(* Logix 5000 AddOnInstructionDefinition export AMP_Hard_Stop_Homing; software revision 20.04 *)

TYPE AMP_Status_Word :   // Applied Motion Input Assembly Status Word
STRUCT
   Enabled : BOOL;   // Motor Enabled (Motor Disabled if this bit = 0)
   Sampling : BOOL;   // Sampling (for Quick Tuner)
   Drive_Fault : BOOL;   // Drive Fault (check Alarm Code)
   In_Position : BOOL;   // In Position (motor is in position)
   Moving : BOOL;   // Moving (motor is moving)
   Jogging : BOOL;   // Jogging (currently in jog mode)
   Stopping : BOOL;   // Stopping (in the process of stopping from a stop command)
   Waiting : BOOL;   // Waiting (for an input; executing a WI command)
   Saving : BOOL;   // Saving (parameter data is being saved)
   Alarm_Present : BOOL;   // Alarm present (check Alarm Code)
   Homing : BOOL;   // Homing (executing an SH command)
   Wait_Time : BOOL;   // Waiting (for time; executing a WD or WT command)
   Wizard_Running : BOOL;   // Wizard running (Timing Wizard is running)
   Checking_Encoder : BOOL;   // Checking encoder (Timing Wizard is running)
   Q_Program_Running : BOOL;   // Q Program is running
   Initializing : BOOL;   // Initializing (happens at power up) ; Servo Ready (for SV200 drives only)
END_STRUCT
END_TYPE

TYPE AMP_Input_Assembly_v2 :   // Applied Motion Drive Input Assembly Version 2.0
STRUCT
   Status_Code : DINT;   // Status Code
   Alarm_Code : DINT;   // Alarm Code
   Voltage : DINT;   // Supply Voltage (x0.1V)
   Current : DINT;   // Actual Current (mA)
   Temp : DINT;   // Drive Temperature (0.1 deg C)
   Encoder_Position : DINT;   // Encoder Position (20,000 counts = 1 shaft turn)
   Absolute_Position : DINT;   // Absolute Position (20,000 counts = 1 shaft turn)
   Position_Error : DINT;   // Position Error (counts)
   Actual_Velocity : DINT;   // Actual Velocity (rev/sec * 240, 0 when no encoder)
   Extended_Inputs : DINT;   // Input Status (Extended)
   Main_Board_Inputs : DINT;   // Input Status (Main board)
   Word11 : DINT;   // Reserved
   Analog_Input_1 : DINT;   // Analog Input 1 (ADC counts, 0=min V, 16383 = max V)
   Analog_Input_2 : DINT;   // Analog Input 2 (ADC counts, 0=min V, 16383 = max V)
END_STRUCT
END_TYPE

ADD_ON_INSTRUCTION AMP_Hard_Stop_Homing   (* revision 1.0 *)
// Applied Motion - Hard Stop Homing AOI
// Help:
// The Hard Stop Homing AOI accepts all the required parameters for SCL commands HV1, HV2, HV3, HA1, HA2, HA3, HL1, HL2, HL3, HC, HD, HO and then sends the HS command to initiate the Hard Stop Homing move.
VAR_IN_OUT
   Input : DINT[14]; {required}   // Drive Input Assembly
   Output : DINT[16]; {required}   // Drive Output Assembly
        [0]   // Command Word
        [1]   // Jog Speed (0.25 rev/min)
        [2]   // Jog Acceleration (10 rev/s/s)
        [3]   // Jog Deceleration (10 rev/s/s)
        [4]   // Point-to-Point Velocity (0.25 rev/min)
        [5]   // Point-to-Point Acceleration (10 rev/s/s)
        [6]   // Point-to-Point Deceleration (10 rev/s/s)
        [7]   // Point-to-Point Distance (Motor steps)
        [9]   // (2x ASCII Letters in 16 lower word)
        [10]   // Data/Register 1
        [11]   // Data/Register 2
END_VAR
VAR_INPUT
   RPI : DINT := 100; {visible}   // Drive Connection Request Packet Interval (milliseconds)
   Start : BOOL; {required}   // Start the Homing
   HV1 : REAL; {required}   // Velocity used while seeking the hard stop (rev/s)
   HV2 : REAL; {required}   // Velocity when moving offset distance set by HO (rev/s)
   HV3 : REAL; {required}   // Velocity when searching for encoder index if desired (rev/s)
   HA1 : REAL; {required}   // Accel used while seeking the hard stop (rev/s/s)
   HA2 : REAL; {required}   // Accel when moving offset distance set by HO (rev/s/s)
   HA3 : REAL; {required}   // Accel when searching for encoder index if desired (rev/s/s)
   HL1 : REAL; {required}   // Decel used while seeking the hard stop (rev/s/s)
   HL2 : REAL; {required}   // Decel when moving offset distance set by HO (rev/s/s)
   HL3 : REAL; {required}   // Decel when searching for encoder index if desired (rev/s/s)
   HC : REAL; {required}   // Hard Stop Current (Amps)
   HD : DINT; {required}   // Hard Stop Fault Delay (ms)
   HO : DINT; {required}   // Home Offset (steps, negative = CCW, positive = CW)
   HS : DINT; {required}   // Hard Stop method (0 = without index, 1 = with index)
END_VAR
VAR_OUTPUT
   Sent : BOOL; {access Read Only, visible}   // All parameter setting and homing commands have been sent to drive
   In_Progress : BOOL; {access Read Only, visible}   // The setting of parameters and/or homing are in progress
   Done : BOOL; {access Read Only, visible}   // Homing Move completed without errors - desired position reached
   Error : BOOL; {access Read Only, visible}   // Homing failed to complete - drive not ready or faulted
   State : DINT := 34; {access Read Only}   // Internal state of progress
END_VAR
VAR
   Loc_StatusCode : AMP_Status_Word;
   Loc_CommandOff_Timer : TIMER;   // Timer to make sure command value was 0 before sending a new command
   Loc_CommandOn_Timer : TIMER;   // Timer to make sure command value is set long enough to be sent to drive
   Loc_Input_Assembly : AMP_Input_Assembly_v2; {access None}
   Loc_Start_ONS : BOOL; {access None}
END_VAR

ROUTINE Logic   (* ladder *)
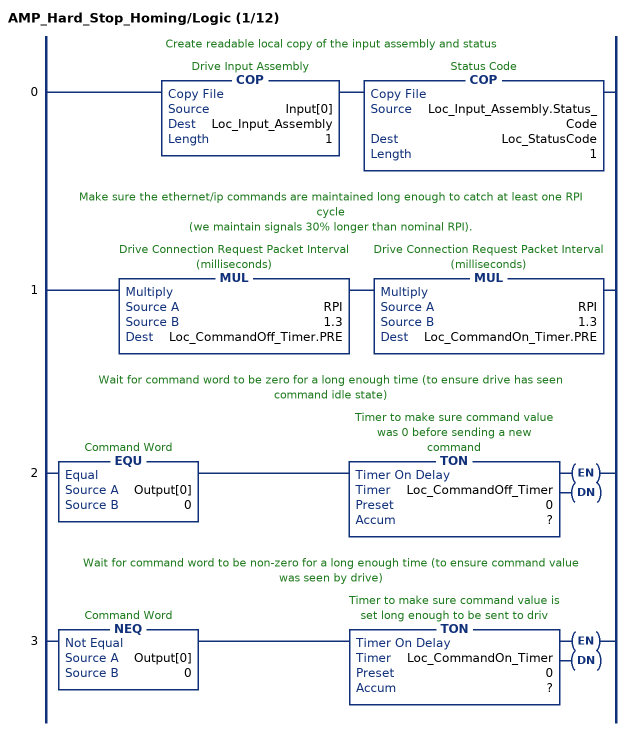
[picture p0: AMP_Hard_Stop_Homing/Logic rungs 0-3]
   // Create readable local copy of the input assembly and status
   0: COP(Input[0],Loc_Input_Assembly,1)COP(Loc_Input_Assembly.Status_Code,Loc_StatusCode,1);
   // Make sure the ethernet/ip commands are maintained long enough to catch at least one RPI cycle
   // (we maintain signals 30% longer than nominal RPI).
   1: MUL(RPI,1.3,Loc_CommandOff_Timer.PRE)MUL(RPI,1.3,Loc_CommandOn_Timer.PRE);
   // Wait for command word to be zero for a long enough time (to ensure drive has seen command idle state)
   2: EQU(Output[0],0)TON(Loc_CommandOff_Timer,?,?);
   // Wait for command word to be non-zero for a long enough time (to ensure command value was seen by drive)
   3: NEQ(Output[0],0)TON(Loc_CommandOn_Timer,?,?);
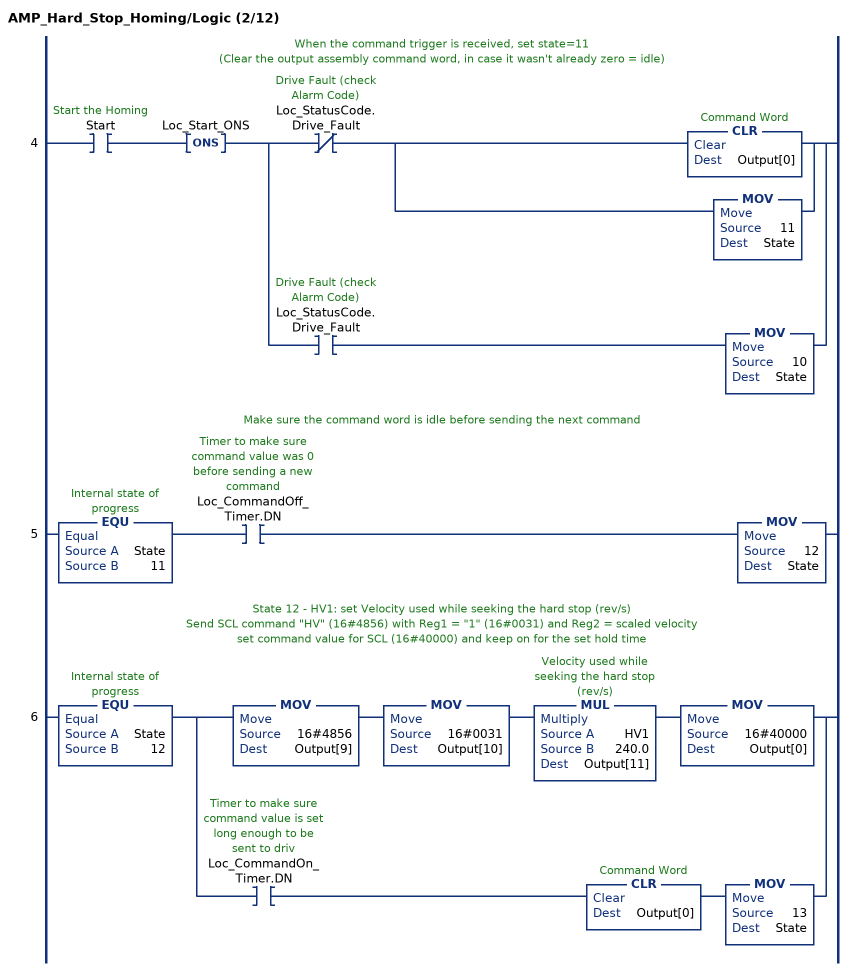
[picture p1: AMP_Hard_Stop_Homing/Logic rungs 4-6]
   // When the command trigger is received, set state=11
   // (Clear the output assembly command word, in case it wasn't already zero = idle)
   4: XIC(Start)ONS(Loc_Start_ONS)[XIO(Loc_StatusCode.Drive_Fault) [CLR(Output[0]) ,MOV(11,State) ] ,XIC(Loc_StatusCode.Drive_Fault) MOV(10,State) ];
   // Make sure the command word is idle before sending the next command
   5: EQU(State,11)XIC(Loc_CommandOff_Timer.DN)MOV(12,State);
   // State 12 - HV1: set Velocity used while seeking the hard stop (rev/s)
   // Send SCL command "HV" (16#4856) with Reg1 = "1" (16#0031) and Reg2 = scaled velocity
   // set command value for SCL (16#40000) and keep on for the set hold time
   6: EQU(State,12)[MOV(16#4856,Output[9]) MOV(16#0031,Output[10]) MUL(HV1,240.0,Output[11]) MOV(16#40000,Output[0]) ,XIC(Loc_CommandOn_Timer.DN) CLR(Output[0]) MOV(13,State) ];
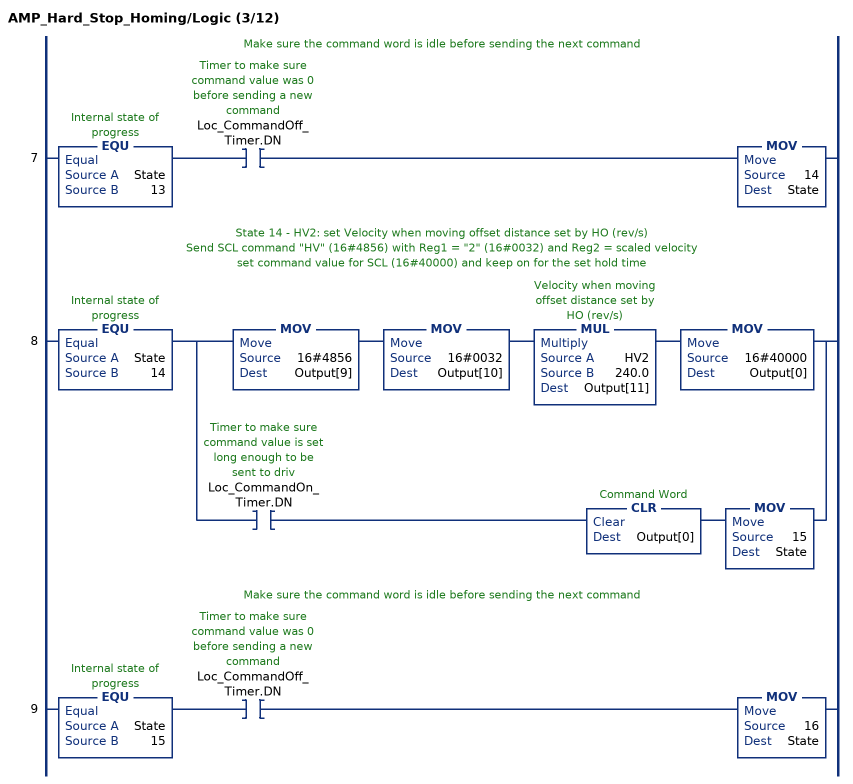
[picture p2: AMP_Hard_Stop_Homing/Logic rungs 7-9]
   // Make sure the command word is idle before sending the next command
   7: EQU(State,13)XIC(Loc_CommandOff_Timer.DN)MOV(14,State);
   // State 14 - HV2: set Velocity when moving offset distance set by HO (rev/s)
   // Send SCL command "HV" (16#4856) with Reg1 = "2" (16#0032) and Reg2 = scaled velocity
   // set command value for SCL (16#40000) and keep on for the set hold time
   8: EQU(State,14)[MOV(16#4856,Output[9]) MOV(16#0032,Output[10]) MUL(HV2,240.0,Output[11]) MOV(16#40000,Output[0]) ,XIC(Loc_CommandOn_Timer.DN) CLR(Output[0]) MOV(15,State) ];
   // Make sure the command word is idle before sending the next command
   9: EQU(State,15)XIC(Loc_CommandOff_Timer.DN)MOV(16,State);
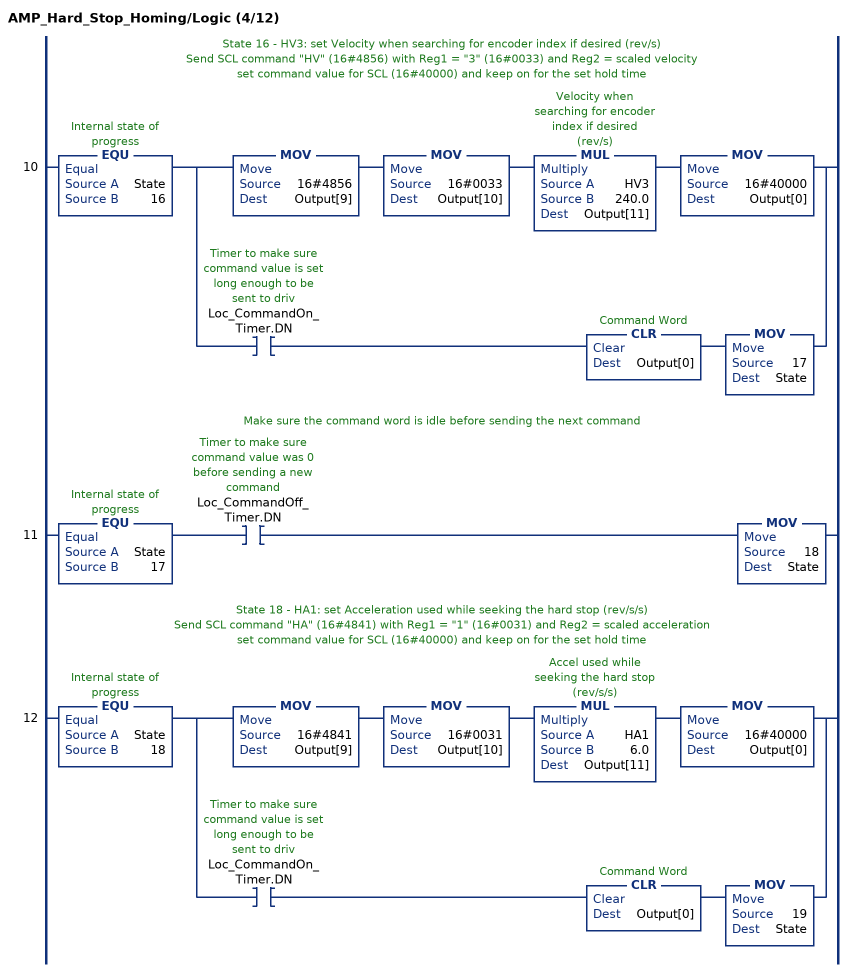
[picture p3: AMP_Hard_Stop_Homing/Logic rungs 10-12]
   // State 16 - HV3: set Velocity when searching for encoder index if desired (rev/s)
   // Send SCL command "HV" (16#4856) with Reg1 = "3" (16#0033) and Reg2 = scaled velocity
   // set command value for SCL (16#40000) and keep on for the set hold time
   10: EQU(State,16)[MOV(16#4856,Output[9]) MOV(16#0033,Output[10]) MUL(HV3,240.0,Output[11]) MOV(16#40000,Output[0]) ,XIC(Loc_CommandOn_Timer.DN) CLR(Output[0]) MOV(17,State) ];
   // Make sure the command word is idle before sending the next command
   11: EQU(State,17)XIC(Loc_CommandOff_Timer.DN)MOV(18,State);
   // State 18 - HA1: set Acceleration used while seeking the hard stop (rev/s/s)
   // Send SCL command "HA" (16#4841) with Reg1 = "1" (16#0031) and Reg2 = scaled acceleration
   // set command value for SCL (16#40000) and keep on for the set hold time
   12: EQU(State,18)[MOV(16#4841,Output[9]) MOV(16#0031,Output[10]) MUL(HA1,6.0,Output[11]) MOV(16#40000,Output[0]) ,XIC(Loc_CommandOn_Timer.DN) CLR(Output[0]) MOV(19,State) ];
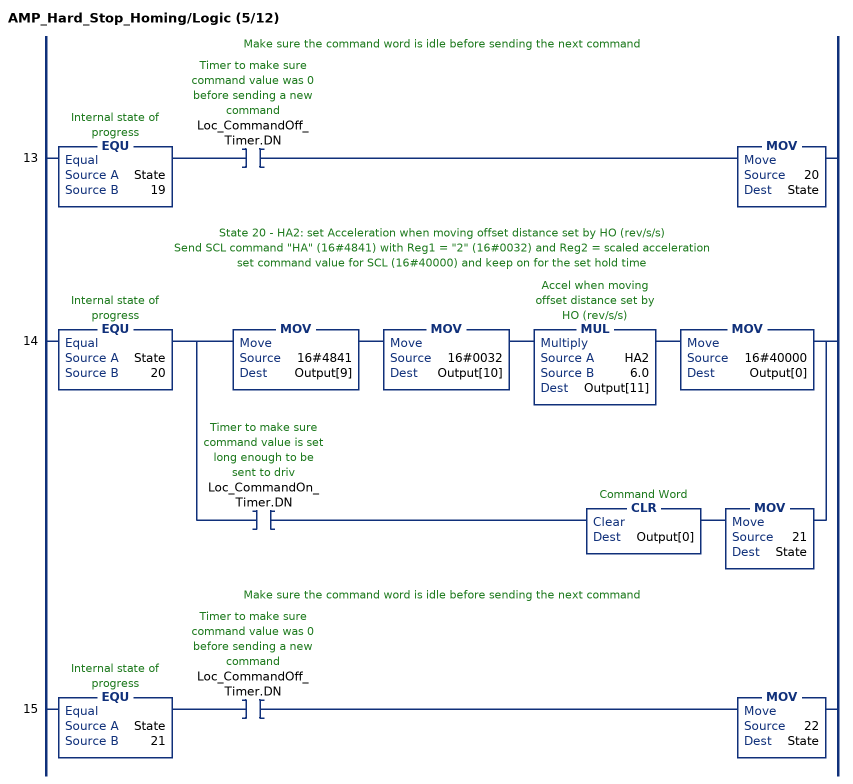
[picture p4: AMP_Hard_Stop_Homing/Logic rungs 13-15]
   // Make sure the command word is idle before sending the next command
   13: EQU(State,19)XIC(Loc_CommandOff_Timer.DN)MOV(20,State);
   // State 20 - HA2: set Acceleration when moving offset distance set by HO (rev/s/s)
   // Send SCL command "HA" (16#4841) with Reg1 = "2" (16#0032) and Reg2 = scaled acceleration
   // set command value for SCL (16#40000) and keep on for the set hold time
   14: EQU(State,20)[MOV(16#4841,Output[9]) MOV(16#0032,Output[10]) MUL(HA2,6.0,Output[11]) MOV(16#40000,Output[0]) ,XIC(Loc_CommandOn_Timer.DN) CLR(Output[0]) MOV(21,State) ];
   // Make sure the command word is idle before sending the next command
   15: EQU(State,21)XIC(Loc_CommandOff_Timer.DN)MOV(22,State);
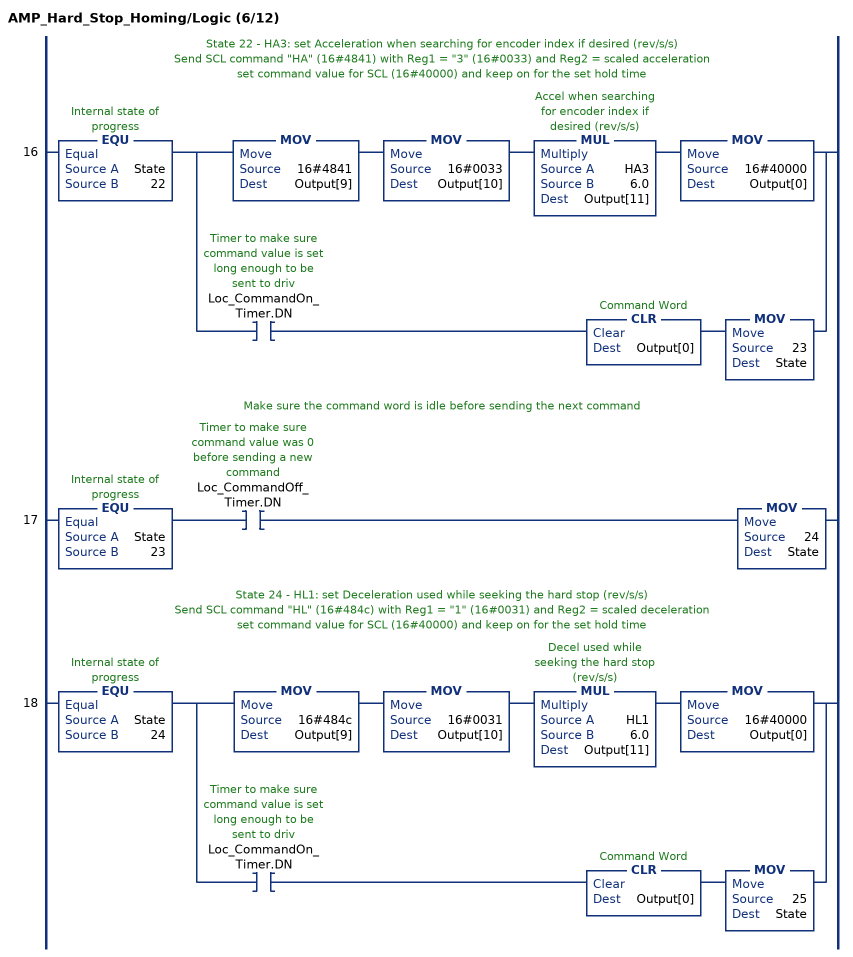
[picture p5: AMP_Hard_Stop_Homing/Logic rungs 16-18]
   // State 22 - HA3: set Acceleration when searching for encoder index if desired (rev/s/s)
   // Send SCL command "HA" (16#4841) with Reg1 = "3" (16#0033) and Reg2 = scaled acceleration
   // set command value for SCL (16#40000) and keep on for the set hold time
   16: EQU(State,22)[MOV(16#4841,Output[9]) MOV(16#0033,Output[10]) MUL(HA3,6.0,Output[11]) MOV(16#40000,Output[0]) ,XIC(Loc_CommandOn_Timer.DN) CLR(Output[0]) MOV(23,State) ];
   // Make sure the command word is idle before sending the next command
   17: EQU(State,23)XIC(Loc_CommandOff_Timer.DN)MOV(24,State);
   // State 24 - HL1: set Deceleration used while seeking the hard stop (rev/s/s)
   // Send SCL command "HL" (16#484c) with Reg1 = "1" (16#0031) and Reg2 = scaled deceleration
   // set command value for SCL (16#40000) and keep on for the set hold time
   18: EQU(State,24)[MOV(16#484c,Output[9]) MOV(16#0031,Output[10]) MUL(HL1,6.0,Output[11]) MOV(16#40000,Output[0]) ,XIC(Loc_CommandOn_Timer.DN) CLR(Output[0]) MOV(25,State) ];
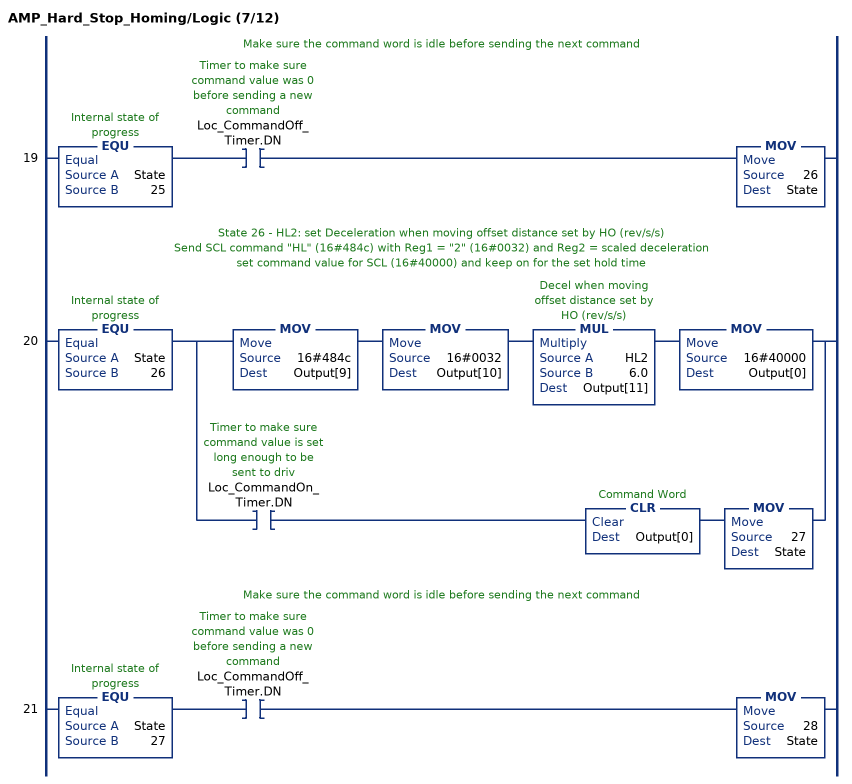
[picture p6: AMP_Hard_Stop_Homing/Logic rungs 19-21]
   // Make sure the command word is idle before sending the next command
   19: EQU(State,25)XIC(Loc_CommandOff_Timer.DN)MOV(26,State);
   // State 26 - HL2: set Deceleration when moving offset distance set by HO (rev/s/s)
   // Send SCL command "HL" (16#484c) with Reg1 = "2" (16#0032) and Reg2 = scaled deceleration
   // set command value for SCL (16#40000) and keep on for the set hold time
   20: EQU(State,26)[MOV(16#484c,Output[9]) MOV(16#0032,Output[10]) MUL(HL2,6.0,Output[11]) MOV(16#40000,Output[0]) ,XIC(Loc_CommandOn_Timer.DN) CLR(Output[0]) MOV(27,State) ];
   // Make sure the command word is idle before sending the next command
   21: EQU(State,27)XIC(Loc_CommandOff_Timer.DN)MOV(28,State);
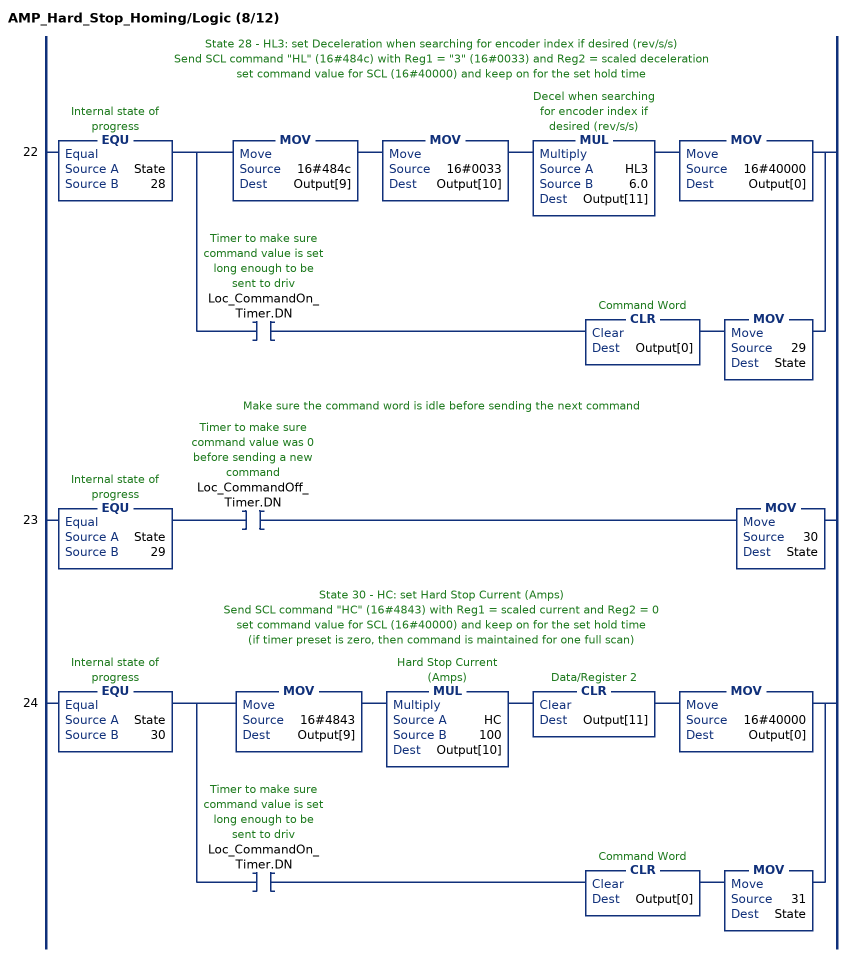
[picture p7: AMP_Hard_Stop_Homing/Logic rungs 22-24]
   // State 28 - HL3: set Deceleration when searching for encoder index if desired (rev/s/s)
   // Send SCL command "HL" (16#484c) with Reg1 = "3" (16#0033) and Reg2 = scaled deceleration
   // set command value for SCL (16#40000) and keep on for the set hold time
   22: EQU(State,28)[MOV(16#484c,Output[9]) MOV(16#0033,Output[10]) MUL(HL3,6.0,Output[11]) MOV(16#40000,Output[0]) ,XIC(Loc_CommandOn_Timer.DN) CLR(Output[0]) MOV(29,State) ];
   // Make sure the command word is idle before sending the next command
   23: EQU(State,29)XIC(Loc_CommandOff_Timer.DN)MOV(30,State);
   // State 30 - HC: set Hard Stop Current (Amps)
   // Send SCL command "HC" (16#4843) with Reg1 = scaled current and Reg2 = 0
   // set command value for SCL (16#40000) and keep on for the set hold time
   // (if timer preset is zero, then command is maintained for one full scan)
   24: EQU(State,30)[MOV(16#4843,Output[9]) MUL(HC,100,Output[10]) CLR(Output[11]) MOV(16#40000,Output[0]) ,XIC(Loc_CommandOn_Timer.DN) CLR(Output[0]) MOV(31,State) ];
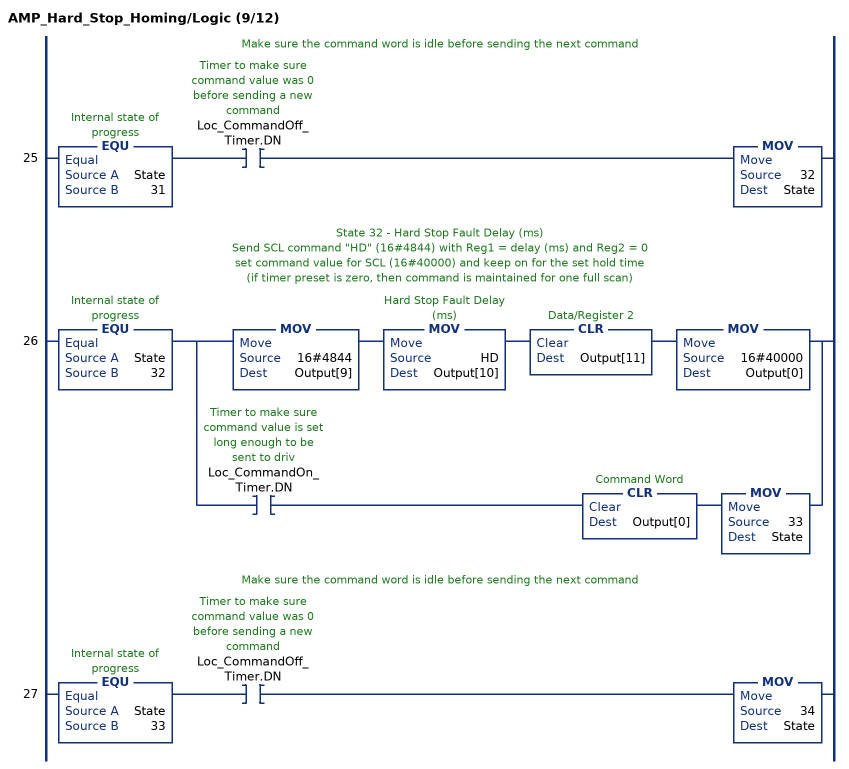
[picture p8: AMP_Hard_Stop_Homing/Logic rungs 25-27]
   // Make sure the command word is idle before sending the next command
   25: EQU(State,31)XIC(Loc_CommandOff_Timer.DN)MOV(32,State);
   // State 32 - Hard Stop Fault Delay (ms)
   // Send SCL command "HD" (16#4844) with Reg1 = delay (ms) and Reg2 = 0
   // set command value for SCL (16#40000) and keep on for the set hold time
   // (if timer preset is zero, then command is maintained for one full scan)
   26: EQU(State,32)[MOV(16#4844,Output[9]) MOV(HD,Output[10]) CLR(Output[11]) MOV(16#40000,Output[0]) ,XIC(Loc_CommandOn_Timer.DN) CLR(Output[0]) MOV(33,State) ];
   // Make sure the command word is idle before sending the next command
   27: EQU(State,33)XIC(Loc_CommandOff_Timer.DN)MOV(34,State);
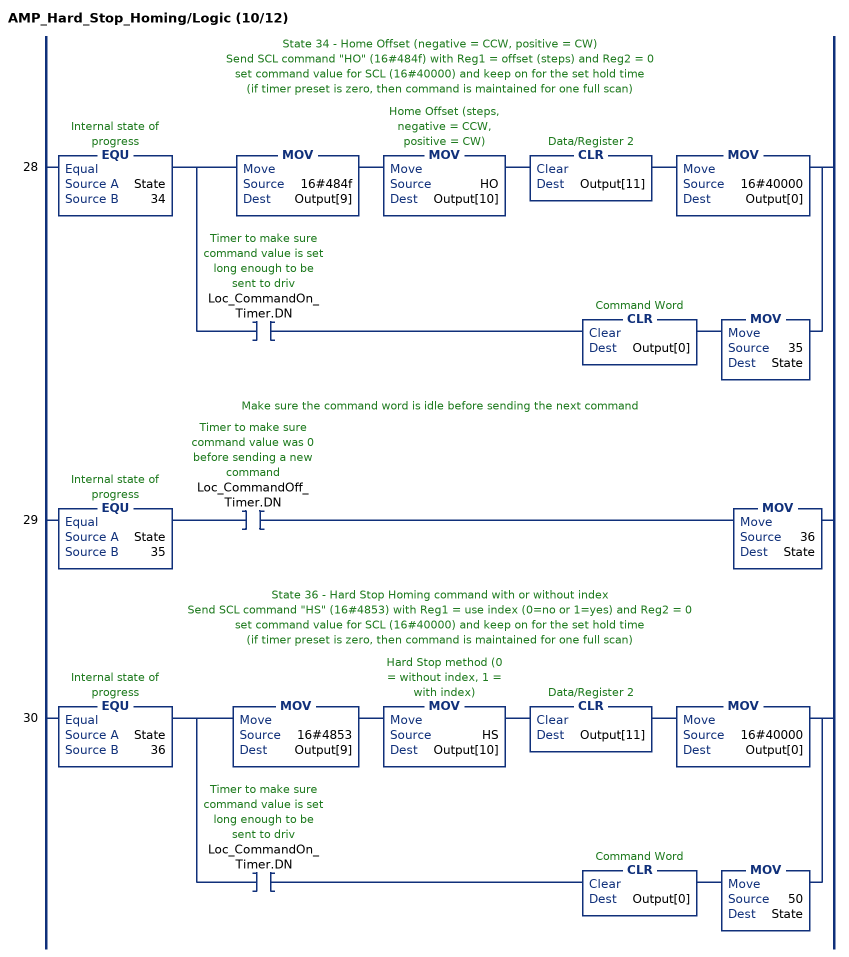
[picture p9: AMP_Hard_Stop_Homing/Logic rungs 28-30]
   // State 34 - Home Offset (negative = CCW, positive = CW)
   // Send SCL command "HO" (16#484f) with Reg1 = offset (steps) and Reg2 = 0
   // set command value for SCL (16#40000) and keep on for the set hold time
   // (if timer preset is zero, then command is maintained for one full scan)
   28: EQU(State,34)[MOV(16#484f,Output[9]) MOV(HO,Output[10]) CLR(Output[11]) MOV(16#40000,Output[0]) ,XIC(Loc_CommandOn_Timer.DN) CLR(Output[0]) MOV(35,State) ];
   // Make sure the command word is idle before sending the next command
   29: EQU(State,35)XIC(Loc_CommandOff_Timer.DN)MOV(36,State);
   // State 36 - Hard Stop Homing command with or without index
   // Send SCL command "HS" (16#4853) with Reg1 = use index (0=no or 1=yes) and Reg2 = 0
   // set command value for SCL (16#40000) and keep on for the set hold time
   // (if timer preset is zero, then command is maintained for one full scan)
   30: EQU(State,36)[MOV(16#4853,Output[9]) MOV(HS,Output[10]) CLR(Output[11]) MOV(16#40000,Output[0]) ,XIC(Loc_CommandOn_Timer.DN) CLR(Output[0]) MOV(50,State) ];
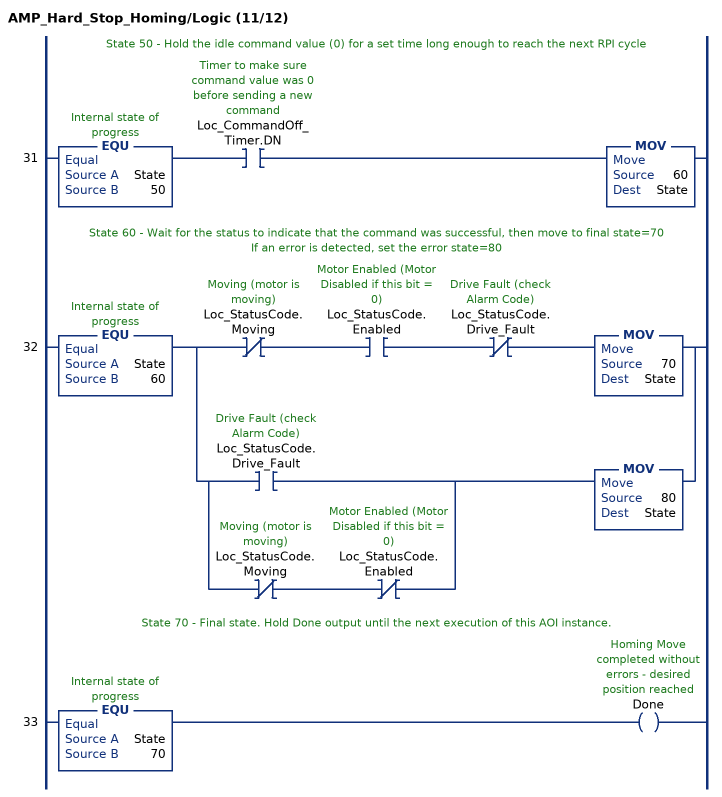
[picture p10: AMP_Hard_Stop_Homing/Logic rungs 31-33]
   // State 50 - Hold the idle command value (0) for a set time long enough to reach the next RPI cycle
   31: EQU(State,50)XIC(Loc_CommandOff_Timer.DN)MOV(60,State);
   // State 60 - Wait for the status to indicate that the command was successful, then move to final state=70
   // If an error is detected, set the error state=80
   32: EQU(State,60)[XIO(Loc_StatusCode.Moving) XIC(Loc_StatusCode.Enabled) XIO(Loc_StatusCode.Drive_Fault) MOV(70,State) ,[XIC(Loc_StatusCode.Drive_Fault) ,XIO(Loc_StatusCode.Moving) XIO(Loc_StatusCode.Enabled) ] MOV(80,State) ];
   // State 70 - Final state. Hold Done output until the next execution of this AOI instance.
   33: EQU(State,70)OTE(Done);
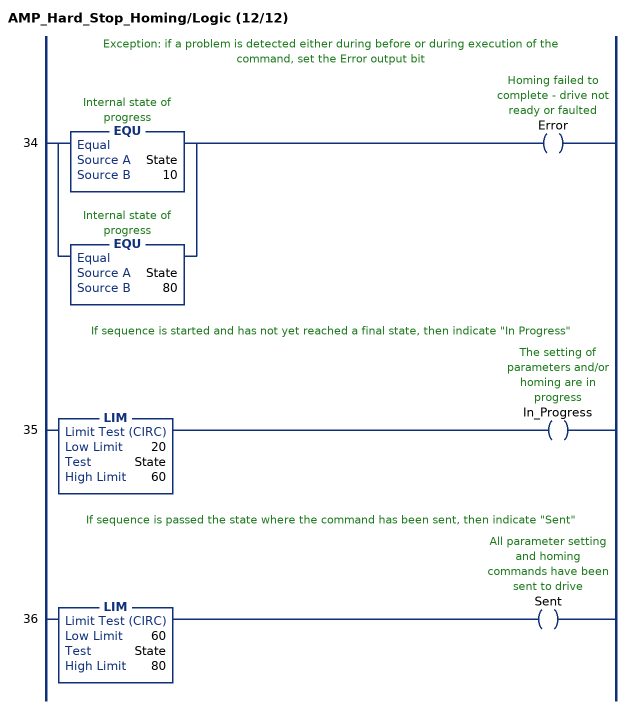
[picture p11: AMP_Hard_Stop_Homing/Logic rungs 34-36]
   // Exception: if a problem is detected either during before or during execution of the command, set the Error output bit
   34: [EQU(State,10) ,EQU(State,80) ]OTE(Error);
   // If sequence is started and has not yet reached a final state, then indicate "In Progress"
   35: LIM(20,State,60)OTE(In_Progress);
   // If sequence is passed the state where the command has been sent, then indicate "Sent"
   36: LIM(60,State,80)OTE(Sent);
END_ROUTINE
END_ADD_ON_INSTRUCTION
